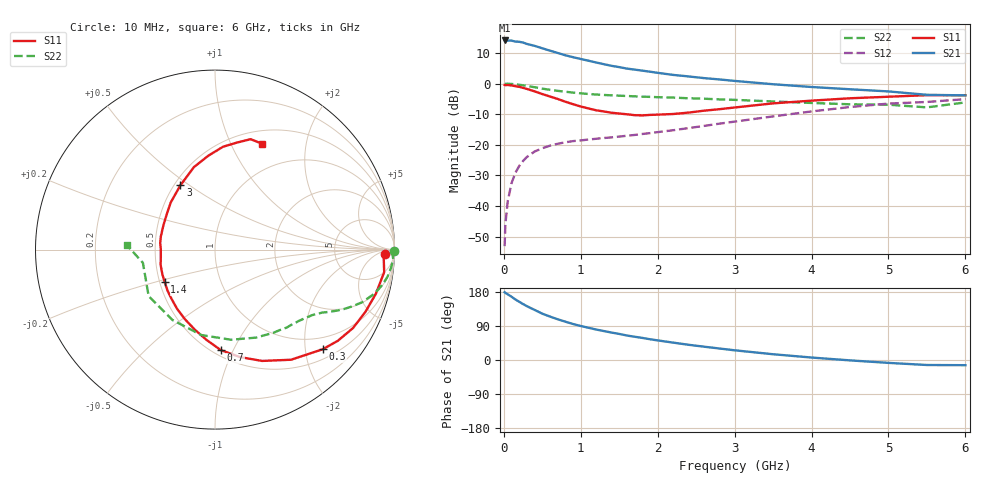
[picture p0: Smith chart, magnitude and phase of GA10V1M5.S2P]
! Infineon Technologies  Discrete & RF Semiconductors
! BF775
! Si NPN RF Bipolar Junction Transistor in SOT23
! VCE = 10 V  IC = 1.5 mA
! Common Emitter S-Parameters:  May  1996
# GHz  S  MA  R  50
!  f  S11  S21  S12  S22
! GHz  MAG  ANG  MAG  ANG  MAG  ANG  MAG  ANG
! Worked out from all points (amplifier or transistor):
!   36 points, 10 MHz to 6 GHz, reference 50 ohm
!   highest |S21| = 14.1 dB at 10 MHz (marker M1)
!   |S21| within 3 dB of that: start of sweep to 556.3 MHz
!   unconditionally stable (mu >= 1): 1.325 GHz to 3.267 GHz
!   at 250 MHz: K = 0.24, MSG = 19.3 dB, |S12| = -25.3 dB
!   at 1.4 GHz: K = 1.04, MAG = 10.5 dB, |S12| = -17.6 dB
!   at 6 GHz: K = 0.95, MSG = 0.6 dB, |S12| = -5.1 dB
!   S11 on the Smith chart (normalised r, x): 10 MHz: 30, -16; 300 MHz: 0.71, -2.37; 700 MHz: 0.55, -0.90; 1.4 GHz: 0.53, -0.22; 3 GHz: 0.54, +0.46; 6 GHz: 0.65, +1.32
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0.01  0.95 -1.6  5.066 178.8  0.0022 91.3  0.9988 -0.5
0.02  0.9414 -3.0  4.935 177.1  0.005 87.5  0.9876 -1.1
0.05  0.9509 -7.6  5.032 173.5  0.0118 84.3  0.9941 -3.0
0.1  0.9297 -15.3  5.037 167.0  0.0236 81.1  0.9861 -5.9
0.15  0.907 -22.5  4.855 159.8  0.0347 76.2  0.9729 -8.9
0.2  0.8846 -29.6  4.821 153.7  0.045 72.7  0.9568 -11.4
0.25  0.8523 -36.6  4.678 147.6  0.0544 68.4  0.9349 -13.9
0.3  0.8174 -42.8  4.442 142.0  0.0632 65.7  0.9144 -16.0
0.4  0.7455 -55.4  4.136 132.2  0.0775 59.6  0.872 -19.6
0.5  0.6734 -67.1  3.77 122.2  0.0877 54.7  0.827 -22.5
0.7  0.5608 -86.7  3.165 107.5  0.1038 48.6  0.7611 -26.5
0.9  0.4599 -104.2  2.699 95.0  0.1147 45.2  0.7121 -29.3
1.1  0.3919 -122.6  2.364 85.1  0.1217 44.1  0.676 -31.9
1.4  0.3337 -147.1  1.95 72.4  0.1319 44.5  0.6426 -35.5
1.7  0.3045 -172.4  1.692 61.4  0.1446 46.4  0.6185 -39.4
2.2  0.3181 154.4  1.386 45.9  0.1726 49.5  0.5903 -47.4
3  0.4065 118.3  1.105 25.6  0.2388 50.8  0.5417 -64.8
3.5  0.4747 104.3  0.975 15.2  0.2907 48.3  0.5101 -79.9
4.5  0.575 85.5  0.807 -1.0  0.4136 37.5  0.4582 -121.2
5  0.6094 78.3  0.744 -7.6  0.4708 29.7  0.4514 -145.0
5.5  0.6464 72.1  0.655 -13.2  0.5005 20.3  0.4083 -169.6
6  0.6454 66.3  0.641 -13.7  0.5568 15.4  0.4924 177.0
